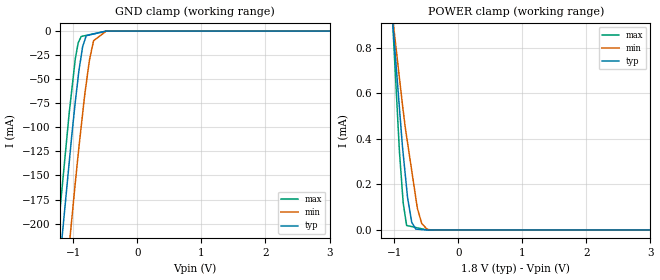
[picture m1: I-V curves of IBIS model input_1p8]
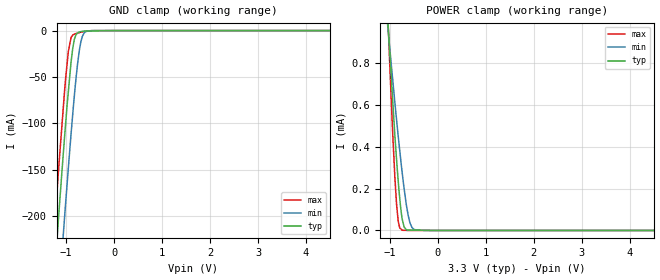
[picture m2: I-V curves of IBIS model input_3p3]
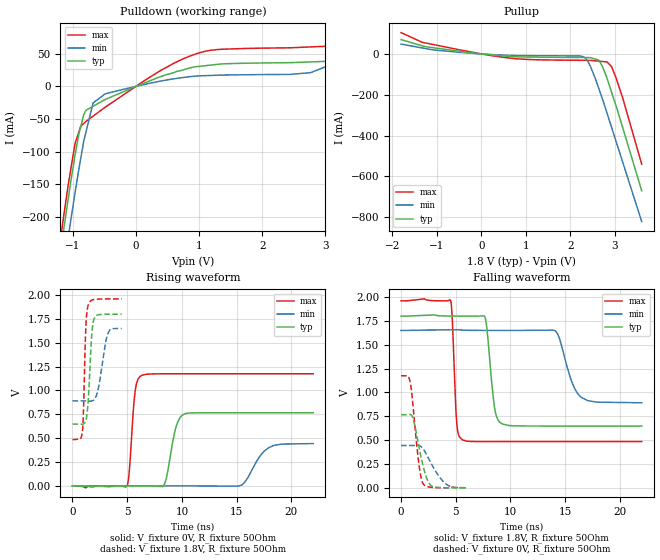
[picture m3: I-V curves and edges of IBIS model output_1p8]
|Texas Instruments Incorporated
| Low-Power, Digital Temperature Sensor with One-Wire Interface
| Marketing part#   Digital Voltage Range   Package-type   #pins
| TMP104YFFR   1.4V - 3.6V   WCSP   4
| TMP104YFFT   1.4V - 3.6V   WCSP   4
[IBIS Ver]   3.2
[File name]   tmp104.ibs
[File Rev]   1.0
[Date]   11/7/2011
[Source]
| Texas Instruments Incorporated.
| Analog-eLab Design Center, HPA
| 12500 TI Blvd
| Dallas, TX -75243
| e-mail: elab_scm_ibis@list.ti.com
[Notes]   Revision History:
| Rev 1.0: 11/7/2011
| - Initial version of the model
| - Model generated from simulations in TISPICE
| - Model matched to SPICE simulation
| - C_comp although listed in numerical order of value are
|   obtained from varying PVT conditions. For PVT conditions for
|   each specific value refer the buffer description under
|   respective [Model]. IBIS model user is responsible for using
|   appropriate C_comp to simulate for Signal Integrity.
| - Model names with a trailing _1p8 contains the model for
|   1.8V [1.65V and 1.96V]. Model names with a trailing _3p3 contains
|   the model for 3.3V [3.0V and 3.6V].
[Disclaimer]
| This model is designed as an aid for customers of Texas Instruments.
| TI and its licensors and suppliers make no warranties, either expressed
| or implied, with respect to this  model, including the warranties of
| merchantability or fitness for a particular purpose. The model is
| provided solely on an "as is" basis. The entire risk as to its quality
| and performance is with the customer.
[Copyright]
 (C) Copyright 2011 Texas Instruments Incorporated.All rights reserved.
|   TMP104
[Component]   TMP104
[Manufacturer]   TI
[Package]   |4 WCSP   -  YFF package
|   typ   min   max
R_pkg   0.00046   0.00046   0.00046
L_pkg   0.04489nH   0.04489nH   0.04489nH
C_pkg   0.09083pF   0.09083pF   0.09083pF
[Pin]  signal_name   model_name   R_pin   L_pin   C_pin
A1   V+   POWER   0.00046   0.04489nH  0.09083pF
A2   GND   GND   0.00046   0.04489nH  0.09083pF
B1   TX   OUTPUT   0.00046   0.04489nH  0.09083pF
B2   RX   INPUT   0.00046   0.04489nH  0.09083pF
|   Model Selectors
[Model Selector] INPUT
input_1p8  1.8V digital input
input_3p3  3.3V digital input
[Model Selector] OUTPUT
output_1p8  1.8V digital output
output_3p3  3.3V digital output
| Models and submodels in the file (4): input_1p8 (Input), input_3p3 (Input), output_1p8 (Output), output_3p3 (Output)
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|   input_1p8 Model
[Model]   input_1p8
Model_type   Input
Vinl = 0.54
Vinh = 1.26
|   typ   min   max
|   (nom PVT)   (fast PVT)   (slow PVT)
|C_comp from frequency sweep method (F=0.001MHz)
|Average
|C_comp   8.255e-13   8.043e-13   8.345e-13
|C_comp from LC tank measurement(L=1nH)
|Average
|Resonant Frequency(Hz)   8.200e+09   8.370e+09   8.140e+09
C_comp   3.771e-13   3.619e-13   3.827e-13
| Where nom  PVT is Nominal Process, 1.8V, 25C
|   Fast PVT is Strong Process,  1.96V, -40C
|   Slow PVT is Weak Process,   1.65V, 125C
[Model Spec]
|Subparameter   typ   min   max
Vinh   1.26   1.155   1.372
Vinl   0.54   0.495   0.588
[Voltage Range]   1.8   1.65   1.96
|Ambient Temperature   25   125   -40
|Junction Temperature
[Temperature Range]   25   125   -40
[Power Clamp Reference]   1.8   1.65   1.96
[GND Clamp Reference]   0   0   0
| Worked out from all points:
|   GND clamp passes 1 mA (typ) near -0.55 V on its own axis
|   POWER clamp passes 1 mA (typ) near -1.04 V on its own axis
[GND Clamp]
|   Voltage   I(typ)   I(min)   I(max)
-1.8V     -682.4mA   -763.5mA   -634.3mA
-1.215V   -243.5mA   -332.8mA   -191.6mA
-1.193V   -227.2mA   -316.7mA   -176.2mA
-1.117V   -174mA     -260.5mA   -122.7mA
-1.064V   -137.1mA   -224mA     -85.64mA
-1.024V   -109.2mA   -196.3mA   -61.89mA
-966.3mV  -72.34mA   -156.4mA   -28.04mA
-876.1mV  -25.77mA   -99.12mA   -5.584mA
-797.4mV  -4.756mA   -54.59mA   -4.469mA
-683.1mV  -3.01mA    -10.03mA   -2.849mA
-488.4mV  -52.6uA    -125.8uA   -89.77uA
3.6V      0A         0A         0A
[POWER Clamp]
|   Voltage   I(typ)   I(min)   I(max)
-1.8V     4.246mA    3.004mA    6.07mA
-1.033V   960.9uA    955.5uA    965.7uA
-1.008V   861.1uA    893.4uA    831.7uA
-919.2mV  542.3uA    672.2uA    354.6uA
-858.5mV  333.9uA    523.5uA    118.2uA
-805.6mV  184.9uA    411.3uA    19.83uA
-790.2mV  141.7uA    382.4uA    18.87uA
-725.4mV  33.67uA    260.4uA    14.83uA
-636.9mV  3.209uA    94.7uA     9.298uA
-569.3mV  1.738uA    28.62uA    5.072uA
-483.4mV  0A         3.224uA    0A
3.6V      0A         0A         0A
|   input_3p3 Model
[Model]   input_3p3
Model_type   Input
Vinl = 0.99
Vinh = 2.31
|   typ   min   max
|   (nom PVT)   (fast PVT)   (slow PVT)
|C_comp from frequency sweep method (F=0.001MHz)
|Average
|C_comp   7.589e-13   7.532e-13   7.702e-13
|C_comp from LC tank measurement(L=1nH)
|Average
|Resonant Frequency(Hz)   8.590e+09   8.770e+09   8.530e+09
C_comp   3.436e-13   3.297e-13   3.485e-13
| Where nom  PVT is Nominal Process, 3.3V, 25C
|   Fast PVT is Strong Process,  3.6V, -40C
|   Slow PVT is Weak Process,   3V, 125C
[Model Spec]
|Subparameter   typ   min   max
Vinh   2.31   2.1   2.52
Vinl   0.99   0.9   1.08
[Voltage Range]   3.3   3   3.6
|Ambient Temperature   25   125   -40
|Junction Temperature
[Temperature Range]   25   125   -40
[Power Clamp Reference]   3.3   3   3.6
[GND Clamp Reference]   0   0   0
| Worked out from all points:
|   GND clamp passes 1 mA (typ) near -0.68 V on its own axis
|   POWER clamp passes 1 mA (typ) near -1.04 V on its own axis
[GND Clamp]
|   Voltage   I(typ)   I(min)   I(max)
-3.3V     -1.844A    -1.917A    -1.802A
-1.267V   -281mA     -369mA     -229.7mA
-1.152V   -197.6mA   -285.4mA   -146.1mA
-1.096V   -157.8mA   -245.7mA   -107.9mA
-1.03V    -112.7mA   -199.4mA   -63.35mA
-954mV    -65.97mA   -148.2mA   -22.6mA
-861.3mV  -18.77mA   -89.62mA   -4.871mA
-825mV    -8.761mA   -68.28mA   -3.893mA
-745.8mV  -1.977mA   -29.79mA   -2.519mA
-660mV    -788.7uA   -6.098mA   -1.397mA
-468mV    -375.4uA   -82.11uA   -49.82uA
6.6V      0A         0A         0A
[POWER Clamp]
|   Voltage   I(typ)   I(min)   I(max)
-3.3V     10.75mA    7.19mA     15.83mA
-1.069V   1.103mA    1.041mA    1.187mA
-1.012V   887.2uA    893.9uA    845.3uA
-946.8mV  644uA      735.3uA    491.9uA
-896.4mV  455.5uA    612.4uA    256.6uA
-860.4mV  338.7uA    529.4uA    125.5uA
-824.4mV  232.2uA    447uA      42.46uA
-741.6mV  53.11uA    273.2uA    1.007uA
-702.9mV  16.92uA    199.7uA    771.7nA
-618mV    2.145uA    71.78uA    255.7nA
-492mV    1.705uA    4.112uA    0A
6.6V      0A         0A         0A
|   output_1p8 Model
[Model]   output_1p8
Model_type   Output
Polarity   Non-Inverting
Vmeas = 0.9
Vref = 0.9
Cref = 2pF
Rref = 50
|   typ   min   max
|   (nom PVT)   (fast PVT)   (slow PVT)
|C_comp from frequency sweep method (F=0.001MHz)
|C_comp   3.465e-12   3.394e-12   3.712e-12
|ON state : BUFFER OUTPUT TURNED HIGH
|C_comp   3.465e-12   3.394e-12   3.712e-12
|OFF state: BUFFER OUTPUT TURNED LOW
|C_comp   3.617e-12   3.613e-12   3.824e-12
|C_comp from LC tank measurement(L=1nH)
|Resonant Frequency(Hz)   4.320e+09   4.480e+09   4.150e+09
C_comp   1.359e-12   1.263e-12   1.472e-12
|ON state : BUFFER OUTPUT TURNED HIGH
|Resonant Frequency(Hz)   4.320e+09   4.480e+09   4.150e+09
|C_comp   1.359e-12   1.263e-12   1.472e-12
|OFF state: BUFFER OUTPUT TURNED LOW
|Resonant Frequency(Hz)   4.910e+09   4.980e+09   4.690e+09
|C_comp   1.052e-12   1.022e-12   1.153e-12
| Where nom  PVT is Nominal Process, 1.8V, 25C
|   Fast PVT is Strong Process,  1.96V, -40C
|   Slow PVT is Weak Process,   1.65V, 125C
[Voltage Range]   1.8   1.65   1.96
|Ambient Temperature   25   125   -40
|Junction Temperature
[Temperature Range]   25   125   -40
[Pullup Reference]   1.8   1.65   1.96
[Pulldown Reference]   0   0   0
[Power Clamp Reference]   1.8   1.65   1.96
[GND Clamp Reference]   0   0   0
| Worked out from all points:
|   slope of the pulldown table from 0 to 0.27 V, typ, clamps not added: 25.9 ohm
|   slope of the pullup table from 0 to 0.27 V, typ, clamps not added: 46.3 ohm
|   falling waveform, V_fixture 1.8V, R_fixture 50Ohm: 20-80 % time 568ps typ, 1.21ns min, 309ps max; typ from 1.8 V to 0.648 V
|   rising waveform, V_fixture 0V, R_fixture 50Ohm: 20-80 % time 745ps typ, 1.41ns min, 431ps max; typ from 0 V to 0.767 V
|   rising waveform, V_fixture 1.8V, R_fixture 50Ohm: 20-80 % time 322ps typ, 621ps min, 219ps max; typ from 0.648 V to 1.8 V
|   falling waveform, V_fixture 0V, R_fixture 50Ohm: 20-80 % time 865ps typ, 1.37ns min, 623ps max; typ from 0.767 V to 0 V
[Pulldown]
|   Voltage   I(typ)   I(min)   I(max)
-1.8V     -673.2mA   -719.8mA   -667.2mA
-1.249V   -285.4mA   -345.2mA   -267.5mA
-1.145V   -217.2mA   -274.5mA   -196.9mA
-1.042V   -149.8mA   -209.5mA   -130.8mA
-968.2mV  -105.3mA   -162.8mA   -87.6mA
-831.6mV  -43.6mA    -84.66mA   -56.91mA
-681.5mV  -30.52mA   -25.36mA   -45.6mA
-488.4mV  -20.04mA   -11.5mA    -31.83mA
976.1mV   30.37mA    15.8mA     50.6mA
3.089V    38.58mA    33.1mA     61.74mA
3.318V    52.79mA    42.84mA    62.69mA
3.6V      70.23mA    54.8mA     88.34mA
[Pullup]
|   Voltage   I(typ)   I(min)   I(max)
-1.8V     70.22mA    48.1mA     104.6mA
-1.325V   39.87mA    29.32mA    56.85mA
252.8mV   -5.468mA   -3.338mA   -9.25mA
1.035V    -15.2mA    -8.68mA    -27.04mA
2.195V    -17.5mA    -10.1mA    -31.16mA
2.343V    -17.78mA   -21.79mA   -31.42mA
2.452V    -18.49mA   -62.12mA   -31.65mA
2.641V    -30.95mA   -171.5mA   -35.53mA
2.822V    -119.3mA   -290.6mA   -39.26mA
2.924V    -187.8mA   -360.1mA   -62.59mA
3.167V    -356.8mA   -526mA     -211.2mA
3.6V      -670.4mA   -821.2mA   -540.1mA
[Ramp]
R_load = 50
|   typ   min   max
dV/dt_r   0.459924/7.41244e-10   0.266287/1.3989e-09   0.704849/4.30094e-10
dV/dt_f   0.691302/5.65474e-10   0.455079/1.21184e-09   0.88498/3.08029e-10
[Falling Waveform]
V_fixture = 1.8V
V_fixture_min = 1.65V
V_fixture_max = 1.96V
R_fixture = 50Ohm
|   Time   V(typ)   V(min)   V(max)
0s        1.8V       1.65V      1.96V
4.532ns   1.801V     1.656V     1.964V
5.096ns   1.8V       1.657V     675.4mV
5.62ns    1.8V       1.654V     502.8mV
7.68ns    1.788V     1.65V      485.2mV
8.536ns   849.4mV    1.65V      485.1mV
9.016ns   687.5mV    1.65V      485mV
14.08ns   647.9mV    1.649V     485mV
16.48ns   647.9mV    947.9mV    485mV
22ns      647.8mV    891.5mV    485mV
[Rising Waveform]
V_fixture = 0V
V_fixture_min = 0V
V_fixture_max = 0V
R_fixture = 50Ohm
|   Time   V(typ)   V(min)   V(max)
0s        295.1pV    1.014nV    238.2pV
5.004ns   -1.26uV    160.9uV    -1mV
5.732ns   -461.1nV   10.2uV     996.3mV
6.348ns   -226.4nV   -5.083uV   1.16V
8.288ns   -3.146mV   -171.9nV   1.175V
9.472ns   622mV      -78.75nV   1.175V
10.26ns   756.6mV    -34.92nV   1.175V
15.48ns   766.5mV    9.371mV    1.175V
17.94ns   766.5mV    401.3mV    1.175V
22ns      766.5mV    443.8mV    1.175V
[Rising Waveform]
V_fixture = 1.8V
V_fixture_min = 1.65V
V_fixture_max = 1.96V
R_fixture = 50Ohm
|   Time   V(typ)   V(min)   V(max)
0s        647.8mV    891.5mV    485mV
700ps     646.8mV    891.6mV    490.2mV
936ps     646.9mV    891.5mV    599.1mV
1.216ns   685.1mV    890.1mV    1.655V
1.468ns   942.9mV    888.1mV    1.905V
1.736ns   1.546V     889.3mV    1.945V
1.944ns   1.741V     901.1mV    1.952V
2.396ns   1.794V     1.042V     1.957V
3.272ns   1.799V     1.606V     1.96V
4.496ns   1.8V       1.65V      1.96V
[Falling Waveform]
V_fixture = 0V
V_fixture_min = 0V
V_fixture_max = 0V
R_fixture = 50Ohm
|   Time   V(typ)   V(min)   V(max)
0s        766.5mV    443.9mV    1.175V
616ps     766.6mV    443.9mV    1.174V
820ps     769mV      443.8mV    1.117V
1.136ns   713.1mV    444mV      812.6mV
1.644ns   426.6mV    444mV      242.7mV
2.016ns   230mV      410.2mV    43.07mV
2.368ns   94.95mV    342.8mV    13.91mV
2.788ns   18.32mV    249.1mV    4.617mV
4.216ns   1.119mV    31.62mV    56.45uV
5.928ns   53.28uV    1.202mV    153.9uV
